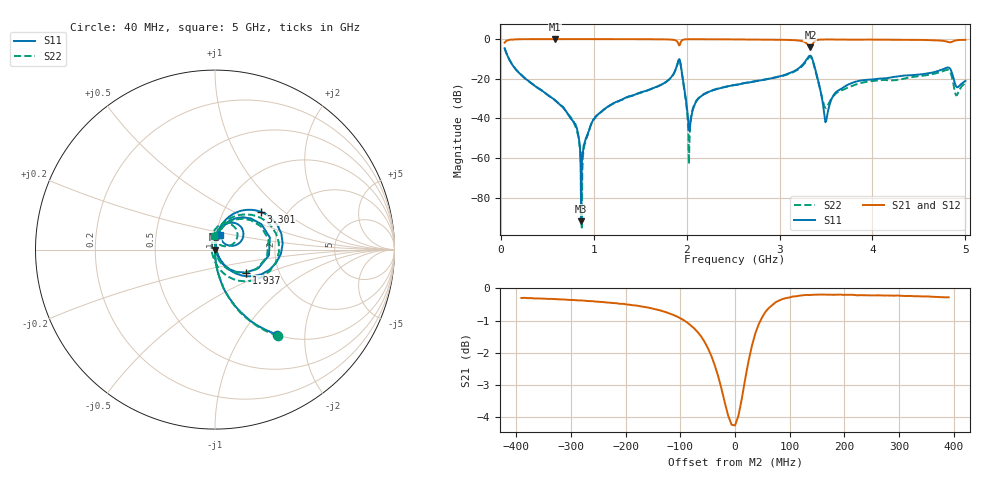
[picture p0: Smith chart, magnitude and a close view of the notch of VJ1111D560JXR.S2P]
! VJ1111D560JXR
! DATE 02/16/2022  11:13
! CAPACITORS MOUNTED IN SERIES ON 25 MIL THICK MICROSTRIP SUBSTRATE
# GHz  S  MA  R  50.00
!  FREQ  S11M  S11A  S21M  S21A  S12M  S12A  S22M  S22A
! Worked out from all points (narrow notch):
!   801 points, 40 MHz to 5 GHz, reference 50 ohm
!   highest |S21| = -0.01 dB at 579.4 MHz (marker M1); lowest = -4.3 dB at 3.332 GHz (marker M2)
!   notch at M2: 4.0 dB deep, 65.5 MHz wide at half that depth
!   lowest |S11| = -92.0 dB at 864.6 MHz (marker M3), VSWR 1.00, Z = 50 - j0.000816 ohm
!   |S11| at or under -10 dB: 86.73 MHz to 3.296 GHz (3.209 GHz wide, 190 % of centre); 3.352 GHz to end of sweep
!   |S22| runs from -95.2 to -4.5 dB; largest |S21 - S12| = 0.038
!   S11 on the Smith chart (normalised r, x): 40 MHz: 1.00, -1.45; 1.937 GHz: 1.36, -0.37; 3.301 GHz: 1.49, +0.70; 5 GHz: 1.04, +0.17
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0.04  0.5857 -54.0  0.8109 35.9  0.8096 35.9  0.5932 -53.9
0.5794  0.02885 -88.8  0.9984 2.6  1.004 2.6  0.02887 -89.6
0.784  0.007936 -82.1  0.9963 1.4  1.004 1.3  0.008162 -93.5
0.8646  2.5e-05 -161.0  0.9965 1.2  1.004 1.0  0.0008545 -101.4
0.8708  0.000695 19.0  0.9972 1.2  1.004 1.0  1.738e-05 -61.0
0.9638  0.006237 89.0  0.9959 0.9  1.004 0.7  0.006587 95.2
1.0444  0.01244 84.7  0.9952 0.7  1.002 0.5  0.01228 88.4
1.6954  0.06529 83.1  0.9861 -1.3  0.9934 -1.6  0.06459 83.9
1.9372  0.2145 -36.7  0.8446 11.9  0.851 11.7  0.2065 -39.5
2.0302  0.004798 21.7  0.9895 2.7  0.9966 2.5  0.003039 91.2
2.1356  0.03322 85.5  0.9894 1.0  0.9965 0.8  0.03372 91.5
2.52  0.06933 83.6  0.9809 -0.7  0.9889 -0.9  0.06979 88.1
3.3012  0.3309 39.5  0.7318 -9.7  0.7369 -9.9  0.3105 34.6
3.3322  0.3786 5.0  0.6128 5.7  0.6175 5.5  0.3565 -2.3
3.3508  0.3227 -20.6  0.7232 16.3  0.7272 16.2  0.3041 -30.1
3.4996  0.008456 22.3  0.9774 4.2  0.9846 4.0  0.01828 178.8
3.5864  0.04009 83.8  0.9749 2.4  0.9827 2.2  0.03808 116.9
3.7104  0.0654 84.8  0.9686 1.2  0.9766 0.9  0.05617 105.9
4.1754  0.105 76.5  0.9619 -0.8  0.9702 -1.0  0.09088 89.3
4.8078  0.1912 44.9  0.8517 -3.2  0.8579 -3.4  0.1666 52.5
4.907  0.06143 36.9  0.9349 3.1  0.9416 2.9  0.03816 60.8
5  0.08783 71.2  0.9549 0.4  0.9612 0.1  0.07804 92.7
